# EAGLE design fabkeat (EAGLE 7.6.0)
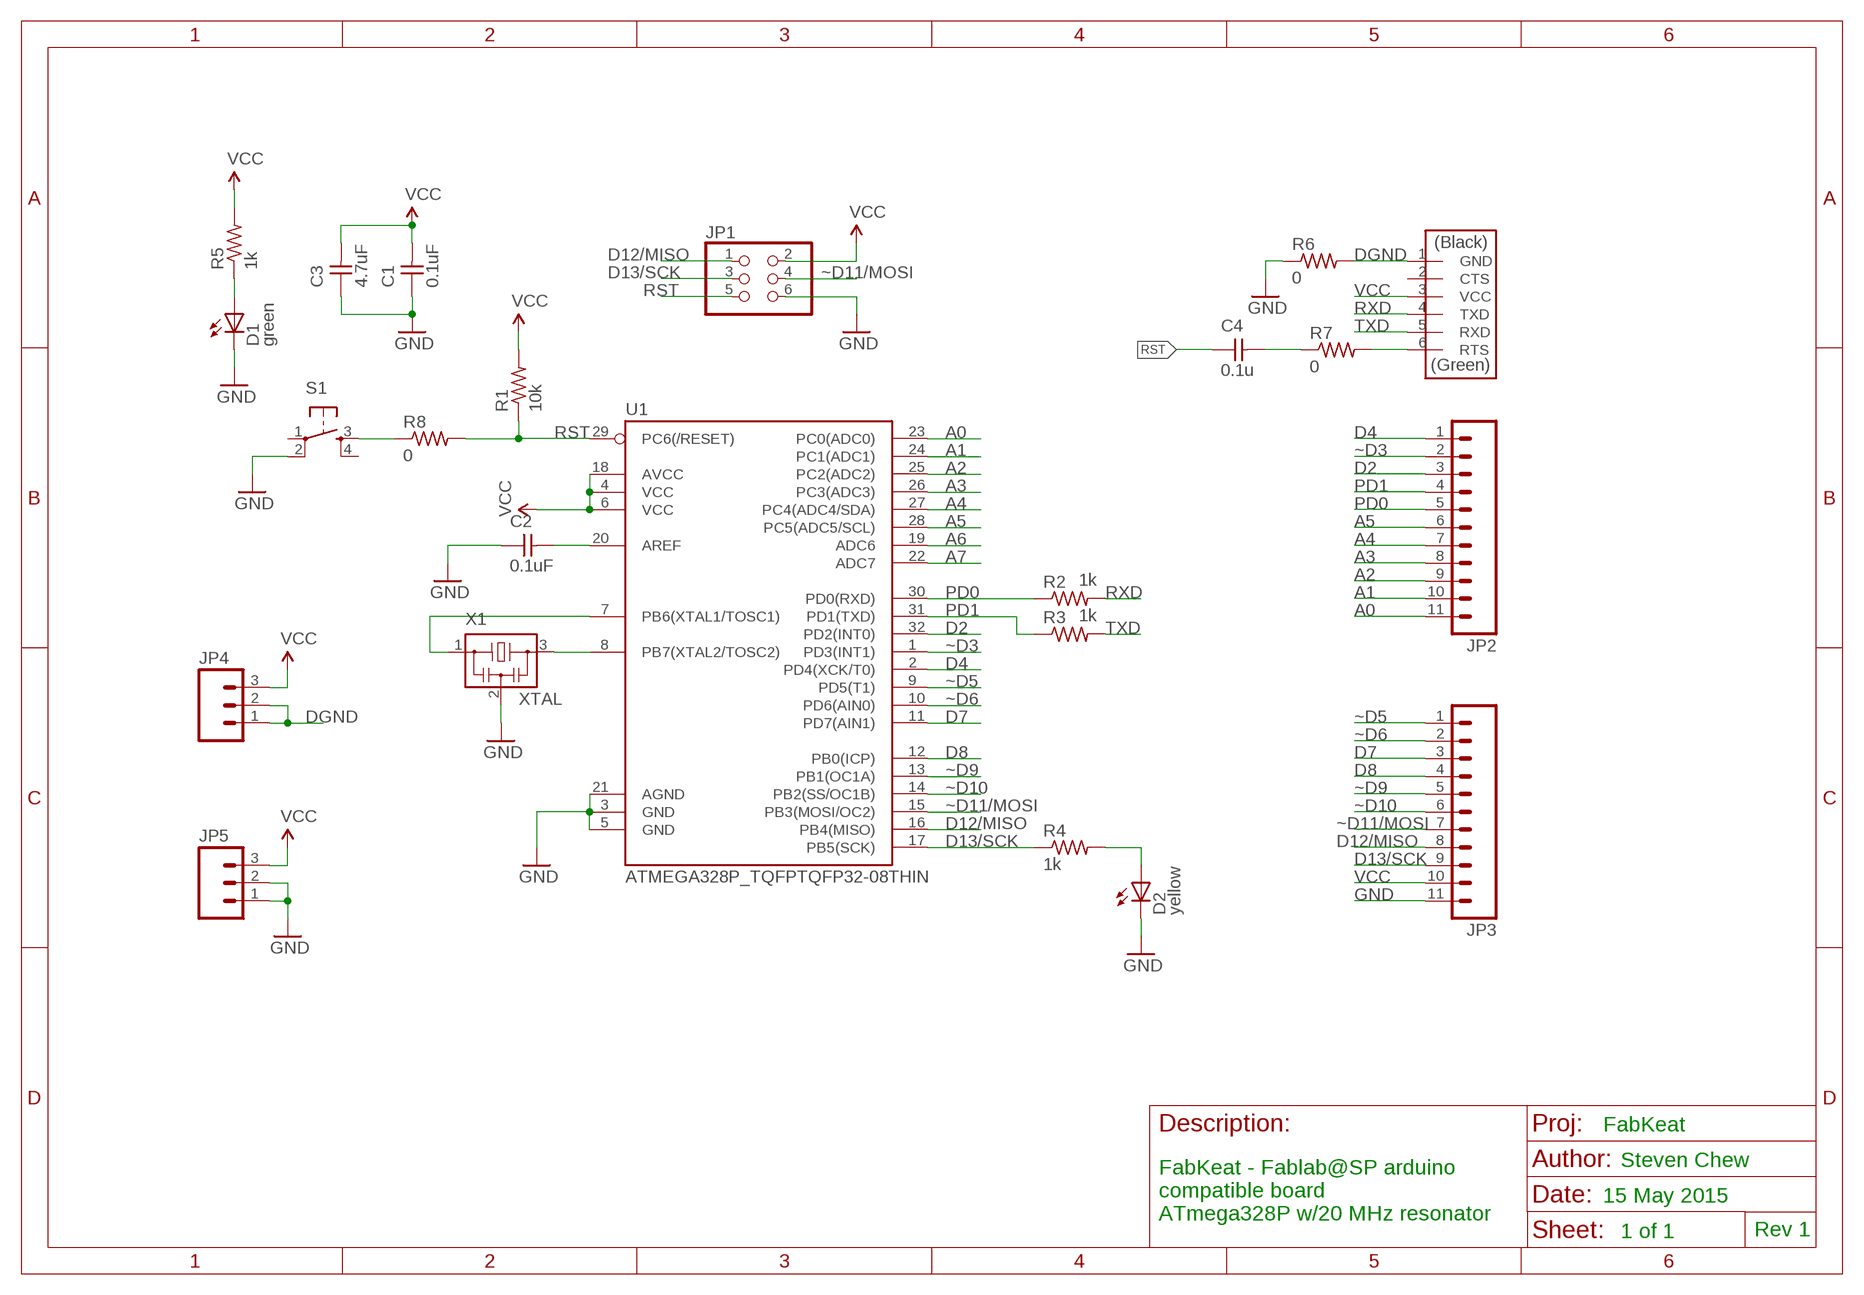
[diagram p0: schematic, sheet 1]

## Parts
C1  0.1uF  CAP-UNPOLARIZEDFAB  [C1206FAB]
C2  0.1uF  CAP-UNPOLARIZED  [C1206]
C3  4.7uF  CAP-UNPOLARIZED  [C1206]
C4  0.1u  CAP-UNPOLARIZEDFAB  [C1206FAB]
D1  green  LEDFAB1206  [LED1206FAB]
D2  yellow  LEDFAB1206  [LED1206FAB]
FTDI  FTDI  FTDI-SMD-HEADER  [1X06SMD]
JP1  PINHD-2X3-SMD  [2X03SMD]
JP2  M11LONGPADS  [1X11_LONGPADS]
JP3  M11LONGPADS  [1X11_LONGPADS]
JP4  M03LONGPADS  [1X03_LONGPADS]
JP5  M03LONGPADS  [1X03_LONGPADS]
R1  10k  RES-US1206FAB  [R1206FAB]
R2  1k  RES-US1206FAB  [R1206FAB]
R3  1k  RES-US1206FAB  [R1206FAB]
R4  1k  RES-US1206FAB  [R1206FAB]
R5  1k  RES-US1206FAB  [R1206FAB]
R6  0  RES-US1206FAB  [R1206FAB]
R7  0  RES-US1206FAB  [R1206FAB]
R8  0  RES-US1206FAB  [R1206FAB]
S1  6MM_SWITCH6MM_SWITCH  [6MM_SWITCH]
U1  ATMEGA328P_TQFPTQFP32-08THIN  [TQFP32-08THIN]
X1  XTAL  RESONATOR  [EFOBM]

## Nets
A0: JP2.11 U1.23(PC0(ADC0))
A1: JP2.10 U1.24(PC1(ADC1))
A2: JP2.9 U1.25(PC2(ADC2))
A3: JP2.8 U1.26(PC3(ADC3))
A4: JP2.7 U1.27(PC4(ADC4/SDA))
A5: JP2.6 U1.28(PC5(ADC5/SCL))
A6: U1.19(ADC6)
A7: U1.22(ADC7)
D2: JP2.3 U1.32(PD2(INT0))
D4: JP2.1 U1.2(PD4(XCK/T0))
D7: JP3.3 U1.11(PD7(AIN1))
D8: JP3.4 U1.12(PB0(ICP))
D12/MISO: JP1.1 JP3.8 U1.16(PB4(MISO))
D13/SCK: JP1.3 JP3.9 R4.1 U1.17(PB5(SCK))
DGND: FTDI.1(GND) JP4.1 JP4.2 R6.2
GND: C1.1 C2.1 C3.1 D1.2(C) D2.2(C) JP1.6 JP3.11 JP5.1 JP5.2 R6.1 S1.2(P1) U1.3(GND) U1.5(GND) U1.21(AGND) X1.2
N$1: D2.1(A) R4.2
N$2: D1.1(A) R5.1
N$3: U1.7(PB6(XTAL1/TOSC1)) X1.1
N$4: U1.8(PB7(XTAL2/TOSC2)) X1.3
N$5: C2.2 U1.20(AREF)
N$6: FTDI.6(RTS) R7.2
N$7: C4.2 R7.1
PD0: JP2.5 R2.1 U1.30(PD0(RXD))
PD1: JP2.4 R3.1 U1.31(PD1(TXD))
RST: C4.1 JP1.5 R1.1 R8.1 R8.2 S1.3(S) U1.29(PC6(/RESET))
RXD: FTDI.4(TXD) R2.2
TXD: FTDI.5(RXD) R3.2
VCC: C1.2 C3.2 FTDI.3(VCC) JP1.2 JP3.10 JP4.3 JP5.3 R1.2 R5.2 U1.4(VCC) U1.6(VCC) U1.18(AVCC)
~D3: JP2.2 U1.1(PD3(INT1))
~D5: JP3.1 U1.9(PD5(T1))
~D6: JP3.2 U1.10(PD6(AIN0))
~D9: JP3.5 U1.13(PB1(OC1A))
~D10: JP3.6 U1.14(PB2(SS/OC1B))
~D11/MOSI: JP1.4 JP3.7 U1.15(PB3(MOSI/OC2))
Unconnected: FTDI.2(CTS) S1.1(P) S1.4(S1)

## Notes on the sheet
- FabKeat
- Steven Chew
- 15 May 2015
- FabKeat - Fablab@SP arduino
  compatible board
  ATmega328P w/20 MHz resonator
- 1 of 1 | Rev 1

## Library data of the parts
C1-C3 = fab:CAP-UNPOLARIZED
C4 = 00fab:CAP-UNPOLARIZED
D1 D2 = fab:LED: LED
FTDI = fab:FTDI-SMD-HEADER
JP1 = fab:PINHD-2X3-SMD: PIN HEADER
JP2 JP3 = SparkFun-Connectors:M11: Header 11 Standard 11-pin 0.1" header. Use with straight break away headers (SKU : PRT-00116), right angle break away headers (PRT-00553), swiss pins (PRT-00743), machine pins (PRT-00117), and female headers (PRT-00115).
JP4 JP5 = SparkFun-Connectors:M03: Header 3 Standard 3-pin 0.1" header. Use with straight break away headers (SKU : PRT-00116), right angle break away headers (PRT-00553), swiss pins (PRT-00743), machine pins (PRT-00117), and female headers (PRT-00115). Molex polarized connector foot print use with SKU : PRT-08232 with associated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
R1-R6 = fab:RES-US: Resistor (US Symbol)
R7 R8 = 00fab:RES-US: Resistor (US Symbol)
S1 = fab:6MM_SWITCH: OMRON SWITCH
U1 = 00fab:ATMEGA328P_TQFP
X1 = fab:RESONATOR

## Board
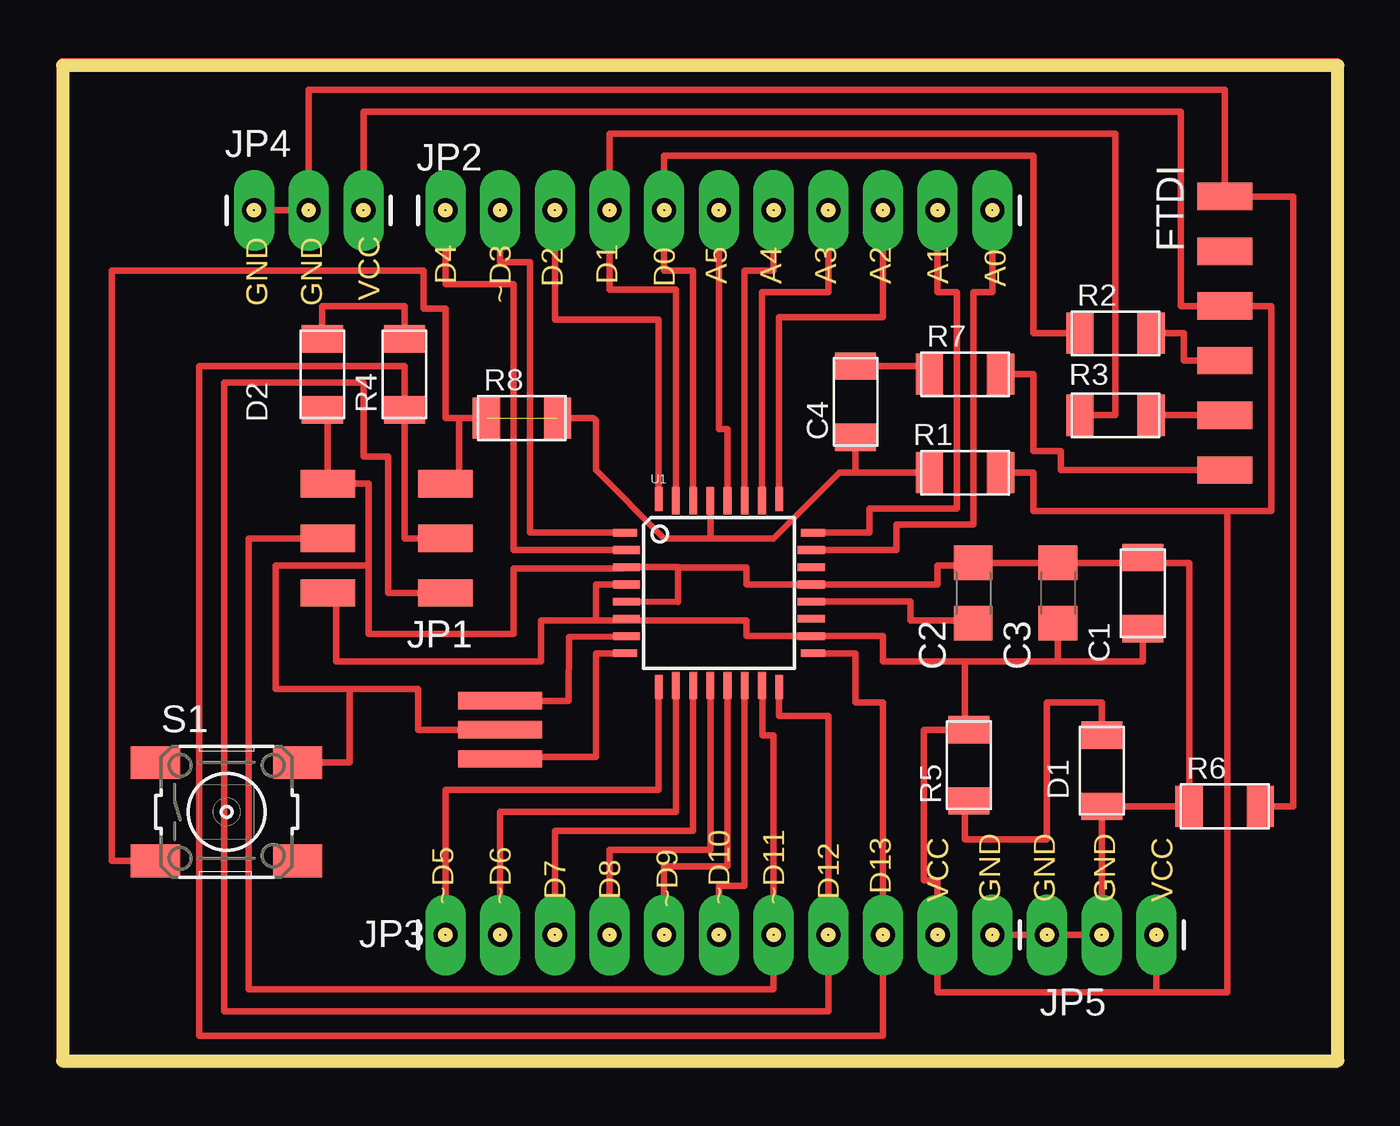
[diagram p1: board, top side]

Size 59.23 x 46.22 mm. Coordinates in mm from the lower left corner, seen from the top.
Outline: 0,0 59.23,0 59.23,46.22 0,46.22 0,0
Outline: circle at 17.78,39.5 radius 0.18
Outline: circle at 20.32,39.5 radius 0.18
Outline: circle at 22.86,39.5 radius 0.18
Outline: circle at 25.4,39.5 radius 0.18
Outline: circle at 27.94,39.5 radius 0.18
Outline: circle at 30.48,39.5 radius 0.18
Outline: circle at 33.02,39.5 radius 0.18
Outline: circle at 35.56,39.5 radius 0.18
Outline: circle at 38.1,39.5 radius 0.18
Outline: circle at 40.64,39.5 radius 0.18
Outline: circle at 43.18,39.5 radius 0.18
Outline: circle at 17.78,5.84 radius 0.18
Outline: circle at 20.32,5.84 radius 0.18
Outline: circle at 22.86,5.84 radius 0.18
Outline: circle at 25.4,5.84 radius 0.18
Outline: circle at 27.94,5.84 radius 0.18
Outline: circle at 30.48,5.84 radius 0.18
Outline: circle at 33.02,5.84 radius 0.18
Outline: circle at 35.56,5.84 radius 0.18
Outline: circle at 38.1,5.84 radius 0.18
Copper layers (1*16): Top 0.035mm / dielectric 1.5mm / Bottom 0.035mm
Design rules "default *": minimum track width 12mil, minimum drill 24mil, track to track 8mil, track to pad 8mil, pad to pad 8mil, via to via 8mil, smd to smd 8mil, copper to edge 40mil, drill to drill 8mil, minimum pad ring 10mil, minimum via ring 8mil, stop-mask expansion 4mil, vias tented up to drill 0mil, thermal gap 10mil

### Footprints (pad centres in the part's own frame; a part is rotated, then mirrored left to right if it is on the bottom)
C1206FAB = smd 1.27 x 1.905: 1 -1.651,0; 2 1.651,0
C1206 = smd 1.6 x 1.8: 1 -1.4,0; 2 1.4,0
LED1206FAB = smd 1.27 x 1.905: 1 -1.651,0; 2 1.651,0
1X06SMD = smd 2.54 x 1.27: 1 0,6.35; 2 0,3.81; 3 0,1.27; 4 0,-1.27; 5 0,-3.81; 6 0,-6.35
2X03SMD = smd 2.54 x 1.27: 1 -2.54,2.54; 2 2.92,2.54; 3 -2.54,0; 4 2.92,0; 5 -2.54,-2.54; 6 2.92,-2.54
1X11_LONGPADS = drill 1.118 pad 1.88 long: 1 0,0; 2 2.54,0; 3 5.08,0; 4 7.62,0; 5 10.16,0; 6 12.7,0; 7 15.24,0; 8 17.78,0; 9 20.32,0; 10 22.86,0; 11 25.4,0
1X03_LONGPADS = drill 1.118 pad 1.88 long: 1 0,0; 2 2.54,0; 3 5.08,0
R1206FAB = smd 1.27 x 1.905: 1 -1.651,0; 2 1.651,0
6MM_SWITCH = smd 2.286 x 1.524: 1 -3.302,2.286; 2 3.302,2.286; 3 -3.302,-2.286; 4 3.302,-2.286
TQFP32-08THIN = smd 1.118 x 0.356: 1 -4.369,2.8; 8 -4.369,-2.8; 17 4.369,-2.8; 24 4.369,2.8 | smd 1.27 x 0.356: 2 -4.293,2; 3 -4.293,1.2; 4 -4.293,0.4; 5 -4.293,-0.4; 6 -4.293,-1.2; 7 -4.293,-2; 18 4.293,-2; 19 4.293,-1.2; 20 4.293,-0.4; 21 4.293,0.4; 22 4.293,1.2; 23 4.293,2 | smd 0.356 x 1.118: 9 -2.8,-4.369; 16 2.8,-4.369; 25 2.8,4.369; 32 -2.8,4.369 | smd 0.356 x 1.27: 10 -2,-4.293; 14 1.2,-4.293; 15 2,-4.293; 26 2,4.293; 27 1.2,4.293; 31 -2,4.293 | smd 0.35 x 1.27: 11 -1.2,-4.293; 12 -0.4,-4.293; 13 0.4,-4.293; 28 0.4,4.293; 29 -0.4,4.293; 30 -1.2,4.293
EFOBM = smd 0.8 x 3.9: 1 -1.35,0; 2 0,0; 3 1.35,0

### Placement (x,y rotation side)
C1  50.16,21.72 270 top
C2  42.29,21.72 270 top
C3  46.23,21.72 270 top
C4  36.83,30.61 90 top
D1  48.26,13.46 270 top
D2  12.06,31.88 270 top
FTDI  53.98,33.78 0 top
JP1  15.24,24.26 180 top
JP2  17.78,39.5 0 top
JP3  17.78,5.84 0 top
JP4  8.89,39.5 0 top
JP5  45.72,5.84 0 top
R1  41.91,27.3 0 top
R2  48.9,33.78 0 top
R3  48.9,29.97 0 top
R4  15.88,31.88 90 top
R5  42.09,13.72 90 top
R6  53.98,11.81 0 top
R7  41.91,31.88 0 top
R8  21.34,29.85 0 top
S1  7.62,11.56 0 top
U1  30.48,21.72 0 top
X1  20.32,15.37 270 top

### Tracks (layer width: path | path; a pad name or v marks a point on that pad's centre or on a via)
A0
  Top 0.305: U1.23 38.73,23.72 38.73,24.89 42.29,24.89 42.29,35.69 43.18,35.69 JP2.11
A1
  Top 0.305: U1.24 37.47,24.52 37.47,25.65 41.53,25.65 41.53,35.69 40.64,35.69 JP2.10
A2
  Top 0.305: JP2.9 38.1,34.54 33.28,34.54 U1.25
A3
  Top 0.305: JP2.8 35.56,35.69 32.48,35.69 U1.26
A4
  Top 0.305: JP2.7 33.02,36.7 31.68,36.7 U1.27
A5
  Top 0.305: JP2.6 30.48,29.34 30.88,29.34 U1.28
D2
  Top 0.305: JP2.3 22.86,34.42 27.69,34.42 27.68,28.07 U1.32
D4
  Top 0.305: U1.2 20.95,23.72 20.95,36.07 17.78,36.07 JP2.1
D7
  Top 0.305: JP3.3 22.86,10.67 29.28,10.67 U1.11
D8
  Top 0.305: JP3.4 25.4,9.78 30.08,9.78 U1.12
D12/MISO
  Top 0.305: JP1.1 15.11,21.72 15.11,28.07 13.97,28.07 13.97,31.5 7.49,31.5 7.49,2.29 35.56,2.29 JP3.8 35.56,16 33.27,16 33.27,17.42 U1.16
D13/SCK
  Top 0.305: JP1.3 15.88,24.26 R4.1 15.88,32.26 6.35,32.26 6.35,1.14 38.1,1.14 JP3.9 38.1,16.64 36.83,16.64 36.83,18.92 U1.17
DGND
  Top 0.305: R6.2 57.15,11.81 57.15,40.13 FTDI.1 53.98,45.09 11.43,45.09 JP4.2 JP4.1
GND
  Top 0.305: 28.57,22.91 28.57,21.31 U1.5 | 28.57,22.91 31.75,22.91 31.75,22.12 U1.21 40.64,22.12 40.64,22.99 42.29,22.99 C2.1 C3.1 50.16,23.12 | 28.57,22.91 28.57,22.92 U1.3 26.06,22.86 20.95,22.86 20.95,19.81 14.22,19.81 14.22,22.99 | D2.2 12.32,30.23 JP1.6 14.22,26.8 14.22,22.99 | 14.22,22.99 9.91,22.99 9.91,17.27 13.34,17.27 | X1.2 16.51,15.37 16.51,17.27 13.34,17.27 | 50.16,23.12 C1.1 | 50.16,23.12 52.32,23.12 R6.1 D1.2 JP5.2 JP5.1 JP3.11 | S1.2 13.34,13.84 13.34,17.27
N$1
  Top 0.305: D2.1 12.06,35.05 15.88,35.05 R4.2
N$2
  Top 0.305: R5.1 41.91,12.06 41.91,10.29 45.72,10.29 45.72,16.64 48.26,16.64 D1.1
N$3
  Top 0.305: X1.1 23.5,16.72 23.52,19.69 26.16,19.71 U1.7
N$4
  Top 0.305: U1.8 24.77,18.92 24.77,14.1 20.32,14.1 X1.3
N$5
  Top 0.305: U1.20 39.37,21.32 39.37,20.45 42.04,20.45 C2.2
N$6
  Top 0.305: R7.2 45.09,31.88 45.09,28.32 46.35,28.32 46.35,27.43 FTDI.6
N$7
  Top 0.305: C4.2 40.26,32.26 R7.1
N$8
  Top 0.406: 0,-0.13 59.18,-0.13 59.18,46.35 0,46.35 0,-0.13
PD0
  Top 0.305: U1.30 29.28,36.7 27.94,36.7 JP2.5 27.94,42.04 45.09,42.04 45.09,33.78 R2.1
PD1
  Top 0.305: U1.31 28.48,35.81 25.4,35.81 JP2.4 25.4,43.05 48.9,43.05 48.9,29.97 R3.1
RST  (1 unrouted)
  Top 0.305: R1.1 36.83,27.3 | 36.83,27.3 36.07,27.3 33.02,24.26 30.1,24.26 | 30.1,24.26 30.1,25.78 U1.29 | JP1.5 18.41,26.8 18.41,29.85 | 30.1,24.26 27.94,24.26 24.77,27.43 24.77,29.72 24.64,29.85 R8.2 | C4.1 36.83,27.3 | R8.1 18.41,29.85 | S1.3 2.29,9.27 2.29,36.7 16.76,36.7 16.76,34.92 17.78,34.92 17.78,29.85 18.41,29.85
RXD
  Top 0.305: R2.2 52.07,33.78 52.07,32.51 FTDI.4
TXD
  Top 0.305: R3.2 FTDI.5
VCC
  Top 0.305: 26.19,20.45 31.75,20.45 31.75,19.72 U1.18 38.1,19.72 38.1,18.54 41.91,18.54 | U1.4 24.77,22.12 24.77,20.45 | 24.77,20.45 26.19,20.45 | 26.19,20.45 U1.6 | JP1.2 12.7,21.72 12.7,18.54 22.23,18.54 22.23,20.45 24.77,20.45 | JP4.3 13.97,44.07 51.94,44.07 51.94,35.05 FTDI.3 56.13,35.05 56.13,25.53 54.1,25.53 | R1.2 45.09,27.3 45.09,25.53 54.1,25.53 | 41.91,18.54 46.23,18.54 | 46.23,18.54 C3.2 | C1.2 50.16,18.54 46.23,18.54 | R5.2 41.91,15.37 | 41.91,15.37 41.91,18.54 | 41.91,15.37 40.01,15.37 40.01,8.38 40.64,8.38 JP3.10 40.64,3.17 50.8,3.17 | 50.8,3.17 JP5.3 | 54.1,25.53 54.1,3.17 50.8,3.17
~D3
  Top 0.305: U1.1 21.72,24.52 21.72,37.08 20.32,37.08 JP2.2
~D5
  Top 0.305: JP3.1 17.78,12.57 27.68,12.57 U1.9
~D6
  Top 0.305: JP3.2 20.32,11.56 28.48,11.56 U1.10
~D9
  Top 0.305: JP3.5 27.94,9.02 30.88,9.02 U1.13
~D10
  Top 0.305: JP3.6 30.48,8.13 31.68,8.13 U1.14
~D11/MOSI
  Top 0.305: JP1.4 8.64,24.26 8.64,3.3 33.02,3.3 JP3.7 33.02,15.11 32.51,15.11 32.51,17.42 U1.15

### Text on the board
Dimension: D4 | D2 | D1 | D0 | A5 | A4 | A3 | A2 | A1 | A0 | GND | GND | VCC | ~D3 | D7 | D8 | D12 | D13 | ~D5 | ~D6 | ~D9 | ~D10 | ~D11 | VCC | GND | GND | GND | VCC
